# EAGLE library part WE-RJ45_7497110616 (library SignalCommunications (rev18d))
Order Code 7497110616 Design THT xBase-T 10/100/1000 Base-T Ports 1x1 +2USB Application Standard USB3.0 Tab Position UP LED (Left-Right) YELLOW-GREEN/OANGE EMI Fingers NO Details see: http://katalog.we-online.de/en/pbs/WE-LAN_RJ45/7497110616? Updated by Yingchun Shan 2016-08-23 2014 (C) Würth Elektronik
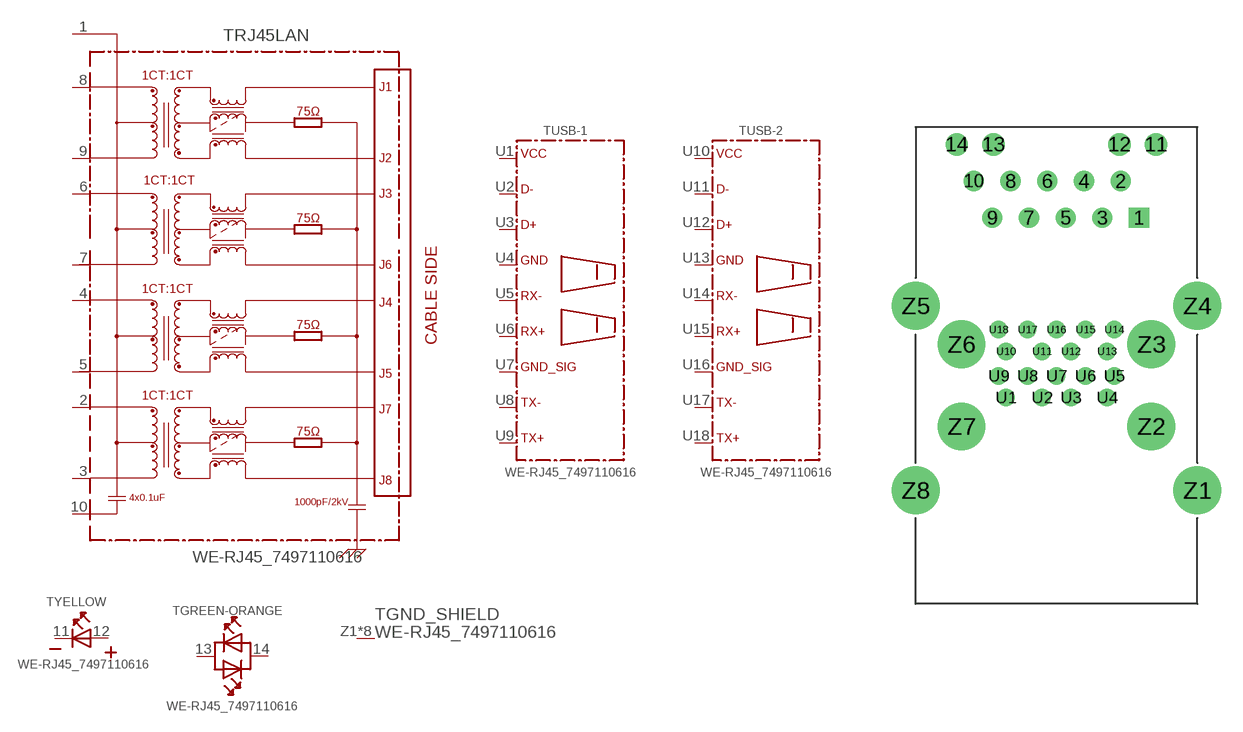
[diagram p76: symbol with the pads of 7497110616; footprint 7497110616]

Designator prefix T; gates RJ45LAN=7497110616 USB-1=USB-3.0 USB-2=USB-3.0 GND_SHIELD=GND_PIN YELLOW=LED-2PIN GREEN-ORANGE=LED-DUAL

## WE-RJ45_7497110616 (COMPANY-URL: http://www.we-online.de; CREATED-BY: Christin Zierenner; CREATED-DATE: AUG 2012; DATASHEET-URL: http://katalog.we-online.de/kataloge/eisos/media/pdf/7497110616.pdf; MANUFACTURER: Würth Elektronik eiSos GmbH)  [7497110616]
1  RJ45LAN:1
2  RJ45LAN:2
3  RJ45LAN:3
4  RJ45LAN:4
5  RJ45LAN:5
6  RJ45LAN:6
7  RJ45LAN:7
8  RJ45LAN:8
9  RJ45LAN:9
10  RJ45LAN:10  pwr
11  YELLOW:K  pas
12  YELLOW:A  pas
13  GREEN-ORANGE:AK1  pas
14  GREEN-ORANGE:AK2  pas
U1  USB-1:VCC  pwr
U2  USB-1:D-
U3  USB-1:D+
U4  USB-1:GND  pwr
U5  USB-1:RX-
U6  USB-1:RX+
U7  USB-1:GND_SIG  pwr
U8  USB-1:TX-
U9  USB-1:TX+
U10  USB-2:VCC  pwr
U11  USB-2:D-
U12  USB-2:D+
U13  USB-2:GND  pwr
U14  USB-2:RX-
U15  USB-2:RX+
U16  USB-2:GND_SIG  pwr
U17  USB-2:TX-
U18  USB-2:TX+
Z1  GND_SHIELD:1  pwr
Z2  GND_SHIELD:1  pwr
Z3  GND_SHIELD:1  pwr
Z4  GND_SHIELD:1  pwr
Z5  GND_SHIELD:1  pwr
Z6  GND_SHIELD:1  pwr
Z7  GND_SHIELD:1  pwr
Z8  GND_SHIELD:1  pwr

## Footprint 7497110616 (pad centres in mm)
incomplete
drill 0.89 square: 1 5.715,18.88
drill 0.89: 2 4.445,21.42; 3 3.175,18.88; 4 1.905,21.42; 5 0.635,18.88; 6 -0.635,21.42; 7 -1.905,18.88; 8 -3.175,21.42; 9 -4.445,18.88; 10 -5.715,21.42
drill 1.03: 11 6.9,23.96; 12 4.36,23.96; 13 -4.36,23.96; 14 -6.9,23.96
drill 0.7: U1 -3.5,6.43; U2 -1,6.43; U3 1,6.43; U4 3.5,6.43; U5 4,7.93; U6 2,7.93; U7 0,7.93; U8 -2,7.93; U9 -4,7.93; U10 -3.5,9.63; U11 -1,9.63; U12 1,9.63; U13 3.5,9.63; U14 4,11.13; U15 2,11.13; U16 0,11.13; U17 -2,11.13; U18 -4,11.13
drill 2.3: Z1 9.75,0; Z2 6.57,4.43; Z3 6.57,10.11; Z4 9.75,12.78; Z5 -9.75,12.78; Z6 -6.57,10.11; Z7 -6.57,4.43; Z8 -9.75,0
